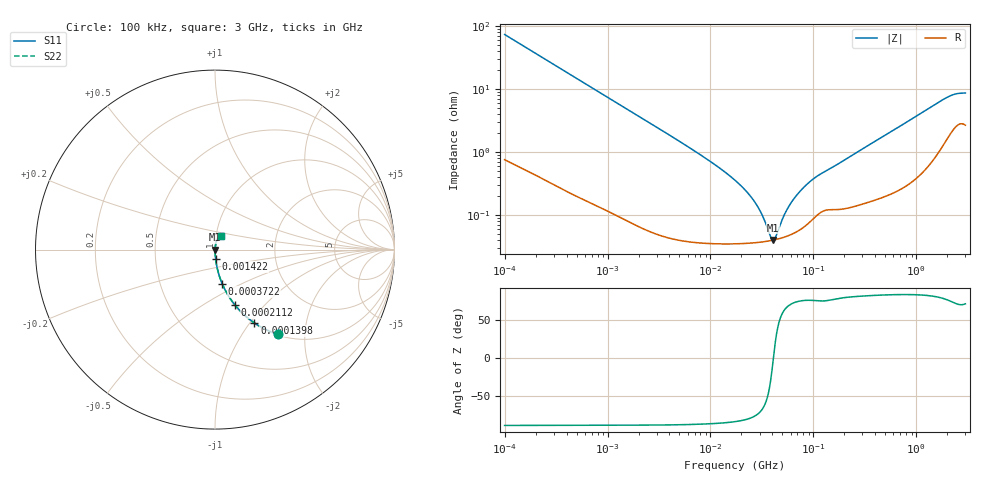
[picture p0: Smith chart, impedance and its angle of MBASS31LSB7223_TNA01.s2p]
! MBASS31LSB7223_TNA01  S-PARAMETER MODEL  ( Standard Model )
! Model Generated by TAIYO YUDEN Corporation (http://www.ty-top.com)
! Version 1.0
! TAIYO YUDEN Control No. 220601
! Copyright(c) 2013 TAIYO YUDEN CO.,LTD. All Rights Reserved.
! Product Description (link to TY-COMPAS)
! https://ds.yuden.co.jp/TYCOMPAS/or/detail?pn=MBASS31LSB7223KTNA01&u=M
! Products Name : Multilayer Ceramic Capacitors
! Characteristics :
!  Capacitance : 0.022 [uF] , Rated Voltage : 630 [V] , TCC : X7R
!  Case Size : 3.2 x 1.6 / 0.126 x 0.063 [mm/inch] , Thickness : 1.6 / 0.063 [mm/inch]
!  (Conditions: Temperature = 25 [degC] , DC Bias Voltage = 0 [V])
! External Node Assignments :
!  1  o---| |---o  2
! GND o---------o GND
! Frequency Range : 100kHz  -  3GHz  [ 401 STEP ]
# MHZ S RI R 50
! Freq[MHz].  S11 Real  S11 Imag  S21 Real  S21 Imag  S12 Real  S12 Imag  S22 Real  S22 Imag
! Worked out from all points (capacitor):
!   401 points, 100 kHz to 3 GHz, reference 50 ohm
!   read as one part in series: C = 21.6 nF near 105.3 kHz
!   lowest |Z| = 40.4 mohm at 40.54 MHz (marker M1)
!   series resonance near 40.89 MHz, so ESL is about 700 pH
!   S11 on the Smith chart (normalised r, x): 100 kHz: 1.02, -1.47; 139.8 kHz: 1.01, -1.05; 211.2 kHz: 1.01, -0.70; 372.2 kHz: 1.01, -0.40; 1.422 MHz: 1.00, -0.11; 3 GHz: 1.05, +0.17
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0.1  0.3518 -0.4724  0.6482 0.4724  0.6482 0.4724  0.3518 -0.4724
0.1398  0.2195 -0.4084  0.7805 0.4084  0.7805 0.4084  0.2195 -0.4084
0.21115  0.1117 -0.3091  0.8883 0.3091  0.8883 0.3091  0.1117 -0.3091
0.372249  0.0404 -0.1905  0.9596 0.1905  0.9596 0.1905  0.0404 -0.1905
0.562235  0.0189 -0.1294  0.9811 0.1294  0.9811 0.1294  0.0189 -0.1294
1.421866  0.00363 -0.0524  0.9964 0.0524  0.9964 0.0524  0.00363 -0.0524
3.161081  0.00104 -0.0236  0.999 0.0236  0.999 0.0236  0.00104 -0.0236
9.574722  0.000412 -0.00744  0.9996 0.00744  0.9996 0.00744  0.000412 -0.00744
17.7727  0.000365 -0.00344  0.9996 0.00344  0.9996 0.00344  0.000365 -0.00344
22.99754  0.000364 -0.00224  0.9996 0.00224  0.9996 0.00224  0.000364 -0.00224
27.54426  0.00037 -0.00149  0.9996 0.00149  0.9996 0.00149  0.00037 -0.00149
32.15051  0.000379 -0.000895  0.9996 0.000895  0.9996 0.000895  0.000379 -0.000895
38.50681  0.000396 -0.000221  0.9996 0.000221  0.9996 0.000221  0.000396 -0.000221
40.54368  0.000403 -3.11e-05  0.9996 3.11e-05  0.9996 3.11e-05  0.000403 -3.11e-05
42.68829  0.000411 0.000159  0.9996 -0.000159  0.9996 -0.000159  0.000411 0.000159
52.46276  0.000452 0.000928  0.9995 -0.000928  0.9995 -0.000928  0.000452 0.000928
61.23616  0.0005 0.00153  0.9995 -0.00153  0.9995 -0.00153  0.0005 0.00153
75.25761  0.000603 0.00238  0.9994 -0.00238  0.9994 -0.00238  0.000603 0.00238
97.38194  0.000857 0.00355  0.9991 -0.00355  0.9991 -0.00355  0.000857 0.00355
547.5153  0.00252 0.0202  0.9975 -0.0202  0.9975 -0.0202  0.00252 0.0202
1935.725  0.0195 0.0682  0.9805 -0.0682  0.9805 -0.0682  0.0195 0.0682
3000  0.0323 0.0779  0.9677 -0.0779  0.9677 -0.0779  0.0323 0.0779
